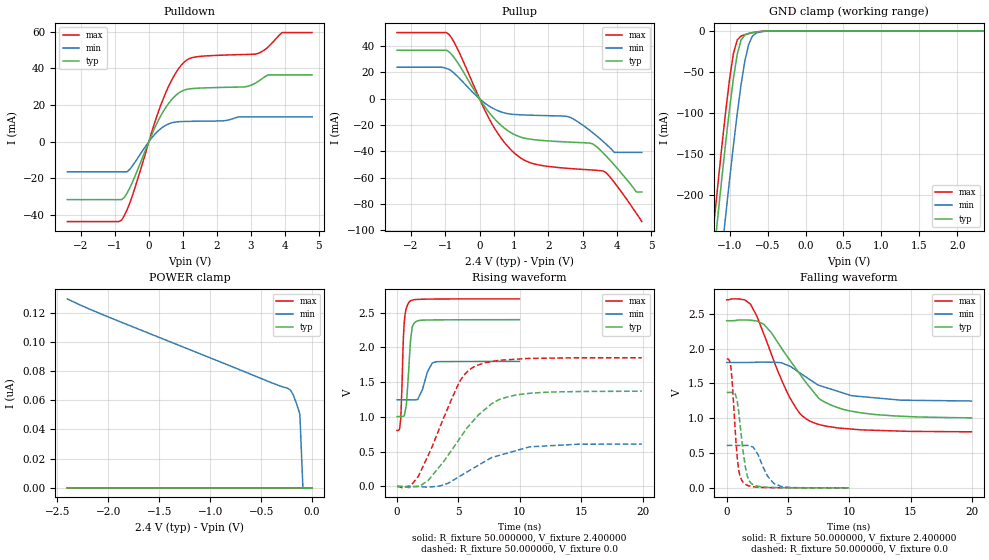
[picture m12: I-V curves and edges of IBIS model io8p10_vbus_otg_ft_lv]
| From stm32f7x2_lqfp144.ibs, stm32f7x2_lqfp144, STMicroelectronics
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|   Model io8p10_vbus_otg_ft_lv
[Model]  io8p10_vbus_otg_ft_lv
Model_type I/O
Polarity   Non-Inverting
Enable   Active-Low
Vinl =   0.720000V
Vinh =   1.680000V
Vmeas =  1.200000V
Cref =   40.000000pF
Rref =   100.000000M
Vref =   0.0V
C_comp   3.193600pF   3.100000pF   3.332100pF
[Temperature Range]   25.000000   0.125000k   -40.000000
[Pullup Reference]   2.400000V   1.800000V   2.700000V
[Pulldown Reference]   0.0V   0.0V   0.0V
[POWER Clamp Reference]   2.400000V   1.800000V   2.700000V
[GND Clamp Reference]   0.0V   0.0V   0.0V
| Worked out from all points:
|   slope of the pulldown table from 0 to 0.36 V, typ, clamps not added: 25 ohm
|   slope of the pullup table from 0 to 0.36 V, typ, clamps not added: 27.7 ohm
|   GND clamp passes 1 mA (typ) near -0.61 V on its own axis
|   rising waveform, R_fixture 50.000000, V_fixture 2.400000: 20-80 % time 311ps typ, 634ps min, 224ps max; typ from 1.01 V to 2.4 V
|   rising waveform, R_fixture 50.000000, V_fixture 0.0: 20-80 % time 3.67ns typ, 4.26ns min, 2.69ns max; typ from 0 V to 1.37 V
|   falling waveform, R_fixture 50.000000, V_fixture 2.400000: 20-80 % time 3.47ns typ, 3.93ns min, 2.74ns max; typ from 2.4 V to 1.01 V
|   falling waveform, R_fixture 50.000000, V_fixture 0.0: 20-80 % time 573ps typ, 1.04ns min, 435ps max; typ from 1.37 V to 0 V
[Pulldown]
|Voltage   I(typ)   I(min)   I(max)
-2.4V     -31.69mA   -16.5mA    -43.66mA
-800mV    -31.69mA   -16.5mA    -42.82mA
-480mV    -21.96mA   -13.17mA   -29.19mA
80mV      3.63mA     1.966mA    5.014mA
480mV     18.16mA    8.738mA    26.02mA
800mV     25.38mA    10.72mA    37.77mA
1.12V     28.53mA    11.02mA    44.6mA
2.8V      29.84mA    13.49mA    47.53mA
3.2V      32.65mA    13.49mA    48.05mA
3.52V     36.43mA    13.49mA    51.84mA
3.92V     36.43mA    13.49mA    59.49mA
4.8V      36.43mA    13.49mA    59.49mA
[Pullup]
|Voltage   I(typ)   I(min)   I(max)
-2.4V     36.91mA    24.04mA    50.37mA
-960mV    36.91mA    23.05mA    50.37mA
-640mV    27.65mA    17.03mA    38mA
320mV     -11.75mA   -6.207mA   -17.08mA
960mV     -26.47mA   -11.82mA   -40.02mA
1.52V     -30.88mA   -12.51mA   -49.05mA
2.56V     -32.88mA   -13.49mA   -52.9mA
3.28V     -34.19mA   -25.52mA   -54.18mA
3.6V      -41.31mA   -32.61mA   -54.99mA
3.92V     -50.32mA   -40.8mA    -63.62mA
4.56V     -70.9mA    -40.8mA    -87.08mA
4.72V     -70.9mA    -40.8mA    -93.4mA
[GND_clamp]
|Voltage   I(typ)   I(min)   I(max)
-2.4V     -1.425A    -1.509A    -1.394A
-1.25V    -311.3mA   -401.9mA   -273.4mA
-1.2V     -265.5mA   -356.1mA   -227.3mA
-1.15V    -220.5mA   -310.9mA   -182mA
-1.1V     -176.4mA   -266.2mA   -138mA
-1.05V    -133.9mA   -222.5mA   -96.06mA
-950mV    -57.51mA   -139mA     -27.35mA
-900mV    -28.55mA   -100.5mA   -11.03mA
-850mV    -11.33mA   -65.67mA   -6.322mA
-750mV    -3.069mA   -16.69mA   -3.425mA
-600mV    -864.6uA   -1.294mA   -852.2uA
2.35V     0A         0A         0A
[POWER_clamp]
|Voltage   I(typ)   I(min)   I(max)
-2.4V     0A         129.4nA    0A
-1.98V    0A         116.5nA    0A
-390mV    0A         71.78nA    0A
-240mV    0A         68.22nA    0A
-210mV    0A         66.81nA    0A
-180mV    0A         62.95nA    0A
-120mV    0A         50.47nA    0A
-90mV     0A         0A         0A
0V        0A         0A         0A
[Ramp]
| variable   typ   min   max
dV/dt_r  0.82206/3.66761n   0.36550/4.25445n   1.11108/2.68619n
dV/dt_f  0.83298/3.46593n   0.33300/3.96618n   1.13646/2.74415n
R_load = 50.000000
[Rising Waveform]
R_fixture= 50.000000
V_fixture= 2.400000
V_fixture_min= 1.800000
V_fixture_max= 2.700000
|time   V(typ)   V(min)   V(max)
0s        1.006V     1.247V     804.6mV
300.3ps   1.006V     1.247V     973mV
520.5ps   1.012V     1.247V     2.145V
600.6ps   1.024V     1.247V     2.379V
760.8ps   1.178V     1.247V     2.566V
1.001ns   1.824V     1.247V     2.655V
1.241ns   2.298V     1.246V     2.681V
1.662ns   2.381V     1.25V      2.691V
2.883ns   2.396V     1.778V     2.697V
9.97ns    2.4V       1.8V       2.699V
[Rising Waveform]
R_fixture= 50.000000
V_fixture= 0.0
V_fixture_min= 0.0
V_fixture_max= 0.0
|time   V(typ)   V(min)   V(max)
0s        170uV      66.54uV    528.1uV
1.121ns   -11.63mV   128.9uV    13.29mV
1.762ns   5.633mV    -1.762mV   154.5mV
2.563ns   92.04mV    -7.452mV   456.7mV
5.045ns   674.8mV    139.7mV    1.49V
6.246ns   952.2mV    265.6mV    1.719V
7.728ns   1.192V     416.7mV    1.797V
9.69ns    1.316V     515mV      1.831V
14.77ns   1.366V     608.2mV    1.851V
19.94ns   1.37V      609mV      1.851V
[Falling Waveform]
R_fixture= 50.000000
V_fixture= 2.400000
V_fixture_min= 1.800000
V_fixture_max= 2.700000
|time   V(typ)   V(min)   V(max)
0s        2.4V       1.8V       2.699V
1.441ns   2.41V      1.8V       2.7V
1.922ns   2.407V     1.801V     2.64V
3.043ns   2.344V     1.805V     2.199V
5.125ns   1.838V     1.748V     1.298V
6.006ns   1.621V     1.643V     1.058V
6.647ns   1.471V     1.568V     969.9mV
7.728ns   1.257V     1.46V      900.1mV
10.01ns   1.105V     1.332V     846.2mV
19.94ns   1.006V     1.247V     804.6mV
[Falling Waveform]
R_fixture= 50.000000
V_fixture= 0.0
V_fixture_min= 0.0
V_fixture_max= 0.0
|time   V(typ)   V(min)   V(max)
0s        1.37V      609mV      1.851V
340.3ps   1.37V      609mV      1.725V
840.8ps   1.26V      608.8mV    464.6mV
1.061ns   952mV      608.6mV    184.7mV
1.381ns   464.6mV    608.9mV    70.14mV
1.702ns   156.6mV    609.3mV    35.36mV
2.302ns   34.19mV    545.2mV    13.16mV
3.323ns   7.716mV    168.7mV    3.637mV
4.464ns   2.218mV    17.93mV    1.575mV
9.97ns    170uV      66.54uV    528.1uV
